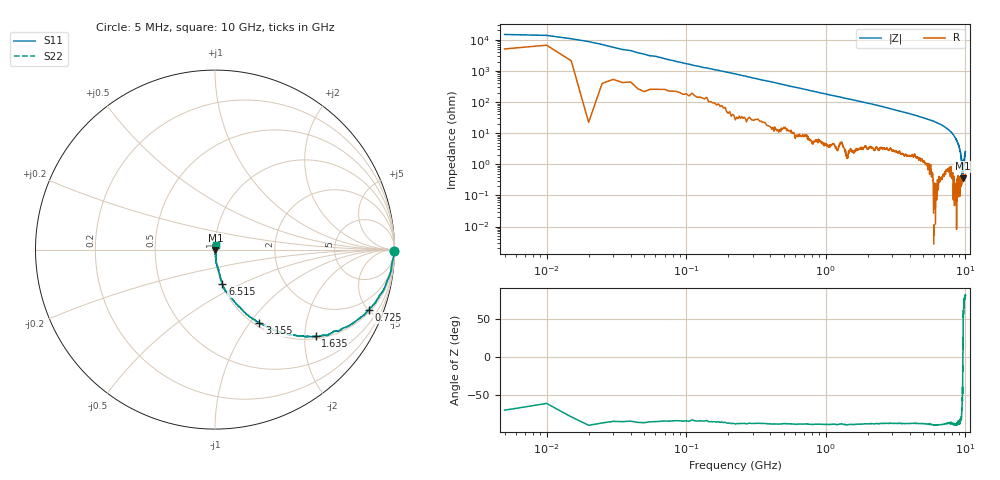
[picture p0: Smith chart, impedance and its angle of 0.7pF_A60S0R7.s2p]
! Amotech Co.,Ltd.
! http://www.amotech.co.kr/
! Part Number: A60S0R7
! These Parameters are Measured in Series Mode Connection
! Operation Temp=25[degC], DC Bias Voltage=0[V]
! Freq. Start=5[MHz] Stop=10[GHz], 2000[Steps]
! Date: Monday, July 13, 2020, 01:47:06
# GHZ S RI R 50.000000
!Freq.(Hz) S11(Real) S11(Imag) S21(Real) S21(Imag) S12(Real) S12(Imag) S22(Real) S22(Imag)
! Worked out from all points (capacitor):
!   2000 points, 5 MHz to 10 GHz, reference 50 ohm
!   read as one part in series: C = 924 fF near 55 MHz
!   lowest |Z| = 357 mohm at 9.545 GHz (marker M1)
!   series resonance near 9.589 GHz, so ESL is about 300 pH
!   S11 on the Smith chart (normalised r, x): 5 MHz: open; 725 MHz: 1.16, -5.02; 1.635 GHz: 1.06, -2.26; 3.155 GHz: 1.05, -1.11; 6.515 GHz: 1.01, -0.40; 10 GHz: 1.01, +0.05
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0.005  0.9977 -0.00628  0.00234 0.00628  0.00234 0.00628  0.9977 -0.00628
0.095  0.9917 -0.0543  0.00834 0.0543  0.00834 0.0543  0.9917 -0.0543
0.195  0.9828 -0.106  0.0172 0.106  0.0172 0.106  0.9828 -0.106
0.385  0.9502 -0.2001  0.0498 0.2001  0.0498 0.2001  0.9502 -0.2001
0.725  0.8555 -0.3364  0.1445 0.3364  0.1445 0.3364  0.8555 -0.3364
1.135  0.7111 -0.4388  0.2889 0.4388  0.2889 0.4388  0.7111 -0.4388
1.635  0.5602 -0.4834  0.4398 0.4834  0.4398 0.4834  0.5602 -0.4834
1.675  0.5504 -0.4843  0.4496 0.4843  0.4496 0.4843  0.5504 -0.4843
3.155  0.2466 -0.4078  0.7534 0.4078  0.7534 0.4078  0.2466 -0.4078
3.34  0.2253 -0.3935  0.7747 0.3935  0.7747 0.3935  0.2253 -0.3935
5.005  0.0978 -0.2771  0.9022 0.2771  0.9022 0.2771  0.0978 -0.2771
6.515  0.0412 -0.1913  0.9588 0.1913  0.9588 0.1913  0.0412 -0.1913
6.67  0.038 -0.1822  0.962 0.1822  0.962 0.1822  0.038 -0.1822
7.85  0.0179 -0.1104  0.9821 0.1104  0.9821 0.1104  0.0179 -0.1104
8.335  0.00731 -0.0779  0.9927 0.0779  0.9927 0.0779  0.00731 -0.0779
8.885  0.00573 -0.0451  0.9943 0.0451  0.9943 0.0451  0.00573 -0.0451
9.21  0.00379 -0.0247  0.9962 0.0247  0.9962 0.0247  0.00379 -0.0247
9.41  0.00353 -0.011  0.9965 0.011  0.9965 0.011  0.00353 -0.011
9.545  0.00265 -0.00238  0.9974 0.00238  0.9974 0.00238  0.00265 -0.00238
9.595  0.00392 1.89e-05  0.9961 -1.89e-05  0.9961 -1.89e-05  0.00392 1.89e-05
9.84  0.00428 0.0151  0.9957 -0.0151  0.9957 -0.0151  0.00428 0.0151
10  0.00467 0.0253  0.9953 -0.0253  0.9953 -0.0253  0.00467 0.0253
